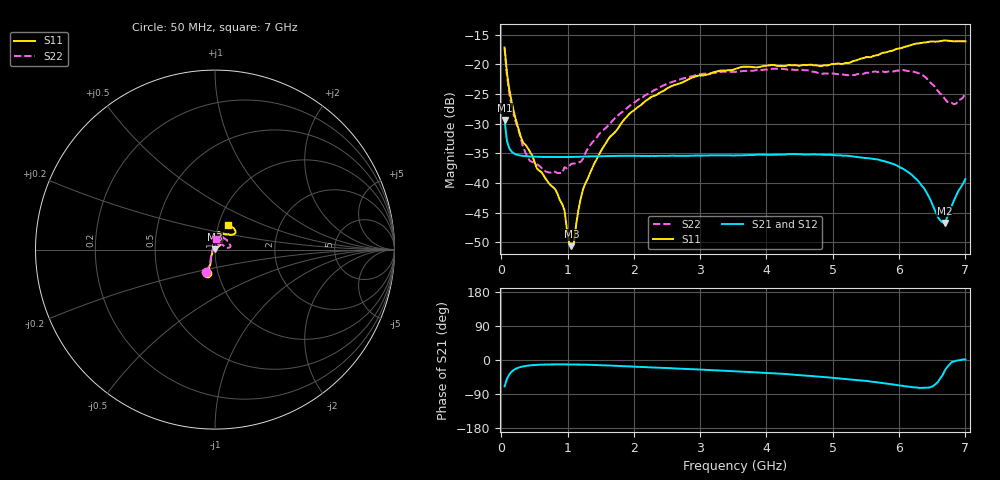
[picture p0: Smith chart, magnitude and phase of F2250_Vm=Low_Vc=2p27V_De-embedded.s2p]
! Integrated Device Technology
! Corporate Headquarters
! 6024 Silver Creek Valley Road
! San Jose, CA 95138  USA
! Phone:  1-408-284-8200
! Toll Free:  1-800-223-1366
! Webpage:  http://www.idt.com/
! Timing and RF Division
! 515 Groton Road, Suite 102
! Westford, MA 01886-6024
! Device:  F2250
! Description: Voltage Variable RF Attenuator
! Frequency:  50.0 -  6000.00 MHz
! Package:  3x3 mm Thin QFN Plastic Package: 16 pin
! Ports:  2 RF, 3 DC
!  Pin  1  = GND
!  Pin  2  = NC
!  Pin  3  = RF1  = Port 1
!  Pin  4  = NC
!  Pin  5  = GND
!  Pin  6  = GND
!  Pin  7  = GND
!  Pin  8  = GND
!  Pin  9  = NC
!  Pin 10  = RF2  = Port 2
!  Pin 11  = NC
!  Pin 12  = GND
!  Pin 13  = GND
!  Pin 14  = VCNTRL
!  Pin 15  = VDD
!  Pin 16  = VMODE
! Vcntrl:  2.270 Volts
! Vmode:  +0.000 Volts
! Vdd:  +3.30  Volts
! Current:  1.178 mA
! Data:  The device was measured on a the F2250 evaluation board which has
!  individual transmission lines to the RF pins.  Data was collected
!  using a calibrated network analyzer.  The evaluation board was
!  de-embedded using a TRL calibration technique.
!  The reference plane is the edge of the package pin.
! Misc:  SN 10
!  Action Tracker AT0258
! Date Measured:  2014-11-26
! Date:  2015-10-15  MJV
! Note:
!  Integrated Device Technology supplies this data as a sample of measured
!  data at the package pin for this product.  Your particular data for this
!  product may vary.
!  Data was taken at 25 degrees C.
!  Integrated Device Technology reserves the right to change this data at anytime.
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# GHz S dB R 50
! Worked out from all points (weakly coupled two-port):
!   201 points, 50 MHz to 7 GHz, reference 50 ohm
!   highest |S21| = -29.40 dB at 50 MHz (marker M1); lowest = -46.8 dB at 6.687 GHz (marker M2)
!   lowest |S11| = -50.7 dB at 1.058 GHz (marker M3), VSWR 1.01, Z = 49.8 + j0.244 ohm
!   |S11| at or under -10 dB: start of sweep to end of sweep
!   |S22| runs from -38.3 to -17.3 dB; largest |S21 - S12| = 6.2e-05
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0.05  -17.18 -108.6  -29.40 -69.6  -29.39 -69.6  -17.34 -110.7
0.08475  -21.45 -107.4  -32.89 -50.2  -32.88 -50.2  -21.84 -109.5
0.15425  -26.23 -116.6  -34.71 -31.0  -34.71 -31.0  -26.99 -121.1
0.29325  -32.19 -127.7  -35.38 -18.4  -35.38 -18.4  -32.48 -135.3
0.3975  -34.08 -141.7  -35.51 -15.0  -35.51 -15.0  -35.71 -158.7
0.6755  -39.40 -163.8  -35.62 -11.9  -35.62 -11.9  -38.08 158.6
0.91875  -43.56 158.1  -35.64 -11.5  -35.64 -11.5  -38.30 129.8
0.9535  -44.63 169.8  -35.63 -11.6  -35.63 -11.5  -37.35 127.9
1.023  -50.04 144.1  -35.63 -11.6  -35.62 -11.6  -37.18 111.7
1.05775  -50.65 123.3  -35.62 -11.7  -35.62 -11.6  -36.76 106.4
1.0925  -50.40 90.1  -35.61 -11.7  -35.61 -11.7  -36.72 101.7
1.162  -44.64 56.9  -35.59 -11.9  -35.59 -11.9  -36.54 90.7
1.2315  -41.11 44.3  -35.57 -12.1  -35.57 -12.1  -35.96 81.0
1.6485  -32.12 42.0  -35.47 -14.7  -35.47 -14.7  -29.88 62.2
2.37825  -24.88 47.4  -35.44 -20.4  -35.43 -20.3  -24.01 55.7
3.525  -20.80 72.5  -35.36 -29.6  -35.36 -29.6  -21.29 74.2
4.7065  -20.17 72.3  -35.17 -42.6  -35.16 -42.6  -21.27 71.9
5.85325  -17.82 40.5  -36.60 -63.3  -36.59 -63.4  -21.20 22.3
6.27025  -16.50 40.1  -39.43 -72.6  -39.44 -72.7  -21.42 9.0
6.68725  -15.99 48.8  -46.75 -28.7  -46.75 -28.1  -25.78 27.9
6.861  -16.13 55.1  -42.16 -1.9  -42.13 -1.8  -26.63 57.9
7  -16.12 63.2  -39.34 1.3  -39.29 1.3  -24.75 83.5
